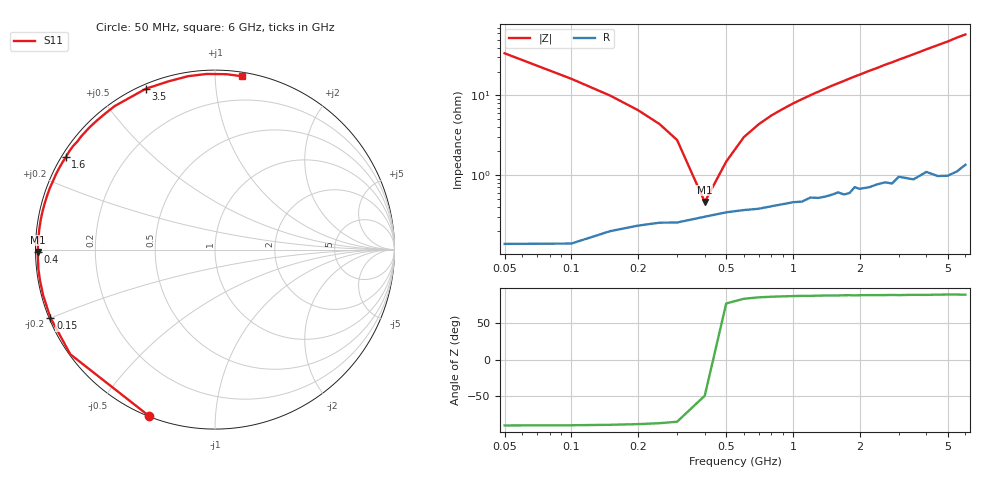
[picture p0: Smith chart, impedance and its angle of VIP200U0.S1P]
! Infineon Technologies  Discrete & RF Semiconductors
! BB 804
! Si Tuning Diode in SOT23
! VR = 0.2 V
! S-Parameters:  July  1999
# GHz  S  MA  R  50
!  f  S11
! GHz  MAG  ANG
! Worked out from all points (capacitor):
!   34 points, 50 MHz to 6 GHz, reference 50 ohm
!   read as one part to ground: C = 92.7 pF near 50 MHz
!   lowest |Z| = 461 mohm at 400 MHz (marker M1)
!   series resonance near 419.5 MHz, so ESL is about 1.6 nH
!   S11 on the Smith chart (normalised r, x): 50 MHz: 0.00, -0.68; 150 MHz: 0.00, -0.20; 400 MHz: 0.01, -0.01; 1.6 GHz: 0.01, +0.28; 3.5 GHz: 0.02, +0.66; 6 GHz: 0.03, +1.17
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0.05  0.9962 -111.8
0.1  0.995 -144.1
0.15  0.9924 -157.5
0.2  0.9909 -165.1
0.25  0.99 -170.0
0.3  0.9899 -173.7
0.4  0.988 -179.2
0.5  0.9865 176.7
0.6  0.9856 173.2
0.8  0.984 167.2
1  0.9823 162.0
1.2  0.9801 157.2
1.5  0.979 150.3
1.6  0.9778 148.2
1.8  0.9787 143.9
1.9  0.975 141.8
2  0.9765 139.9
2.2  0.9761 135.8
2.4  0.9747 132.2
2.6  0.974 128.2
2.8  0.9756 124.9
3  0.9714 121.3
3.5  0.9756 113.3
4  0.9725 105.6
4.5  0.9778 98.8
5  0.9796 92.7
5.5  0.9793 86.3
6  0.9774 81.2
